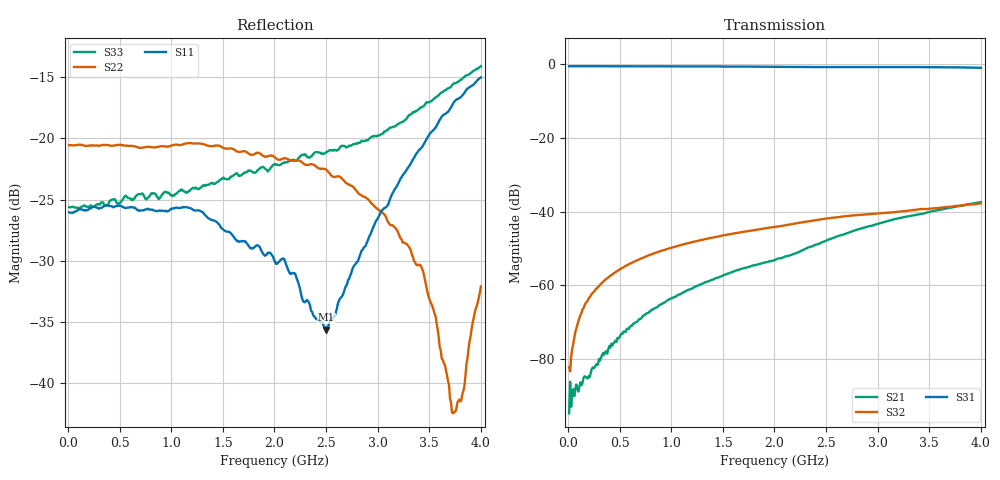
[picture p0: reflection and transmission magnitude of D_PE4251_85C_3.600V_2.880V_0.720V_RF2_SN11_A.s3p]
! Device ID: PE4251_SoldCshunt_081809
! Dir: c:\Test Bench Repositories\Bench_Software_CVI_Version_8\trunk\PSC 4Port_VNA Bench\datalog\4250\TEST\PE4251_SoldCshunt_081809\85C\3p600000\RF2
! Serial: 11
! Insertion: A
! Temp: 85C
! VDD: 3.600
! Control_Hi: 80.000
! Control_Lo: 20.000
! Logic State: RF2
! Port 1: RFC
! Port 2: RF1
! Port 3: RF2
! V1 = 0.72
! V2 = 0.72
! V3 = 0.72
! IDD: 4.958580e-05
! FILE NAME
! DATE 08/18/09  20:17
! CORRECTED  DATA
#  Hz  S  RI  R  50.00
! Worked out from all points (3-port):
!   401 points, 10 MHz to 4 GHz, reference 50 ohm
!   strongest paths, dB at 10 MHz, 1.008 GHz, 2.005 GHz, 3.002 GHz, 4 GHz:
!     S31: -0.6, -0.7, -0.8, -0.8, -1.1
!     S32: -82.2, -49.7, -44.1, -40.5, -37.8
!     S21: -94.6, -63.4, -53.1, -43.3, -37.5
!   lowest |S11| = -35.6 dB at 2.504 GHz (marker M1), VSWR 1.03, Z = 50.4 - j1.6 ohm
!   |S11| at or under -10 dB: start of sweep to end of sweep
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1e7  0.0499 -0.000671  2.73e-05 -1.29e-05  0.9302 -0.00385
     -1.77e-05 5.56e-06  0.0938 -0.001  -7.44e-06 -1.45e-05
     0.9317 -0.00446  7.15e-05 3.07e-05  0.0524 0.000463
1.59625e8  0.0507 0.000204  1.85e-05 -5.35e-05  0.9286 -0.0561
           1.22e-05 -5.74e-05  0.0932 -0.00354  5.67e-05 0.000533
           0.93 -0.0561  6.61e-05 0.000531  0.0533 0.000628
3.0925e8  0.0519 -0.00146  -3.16e-05 -8.84e-05  0.9236 -0.1089
          -4.31e-05 -8.57e-05  0.0931 -0.0081  8.24e-05 0.00102
          0.9242 -0.1081  9.26e-05 0.00102  0.0536 -0.00272
4.78825e8  0.0529 -0.00337  -0.000131 -0.000136  0.9133 -0.1661
           -0.000134 -0.000141  0.0932 -0.0121  0.000145 0.00156
           0.9136 -0.1653  0.000138 0.00157  0.054 -0.00572
9.77575e8  0.0491 -0.0123  -0.000628 -0.000161  0.8675 -0.3267
           -0.000623 -0.000161  0.0894 -0.0253  0.000412 0.00315
           0.8685 -0.326  0.000408 0.00314  0.0583 -0.0142
2.005e9  0.0304 -0.0072  -0.00221 -6.57e-05  0.6858 -0.6034
         -0.00221 -6.25e-05  0.077 -0.0325  0.00104 0.00611
         0.6871 -0.603  0.00104 0.00613  0.0688 -0.0382
2.50375e9  0.00442 -0.0159  -0.00403 -0.000387  0.5755 -0.7006
           -0.00404 -0.000392  0.0681 -0.0297  0.00138 0.00791
           0.5773 -0.7  0.00139 0.00793  0.0506 -0.072
3.42145e9  -0.0825 -0.0394  -0.00906 0.00196  0.3243 -0.8441
           -0.00906 0.00194  0.0242 -0.0177  0.00203 0.0106
           0.3275 -0.8446  0.00203 0.0106  -0.0358 -0.1288
3.74065e9  -0.1356 -0.0392  -0.011 0.00354  0.2144 -0.8702
           -0.011 0.00348  -0.000958 -0.00753  0.00191 0.0116
           0.2147 -0.8703  0.00192 0.0117  -0.0923 -0.1408
4e9  -0.1751 -0.0309  -0.0124 0.00509  0.1189 -0.8795
     -0.0124 0.00503  -0.0247 -0.00232  0.00199 0.0127
     0.1206 -0.8777  0.00198 0.0128  -0.1415 -0.1379
